ORGANIZATION_BLOCK MAIN:OB1
TITLE=Semaforo Pedonale
//Simulatore: 16
//Versione:1.0
//Data 02/03/2002
//------- Descrizione dell'impianto -----------------
//In prossimità di un passaggio pedonale si trova un
//semaforo. Premendo uno dei pulsanti di richiesta SB1 o SB2 da
//parte dei pedoni il semaforo segnala allo scadere di tempi
//prefissati la seguente sequenza sequenza:
// - verde per auto, rosso per pedoni
// - giallo per auto, rosso per pedoni
// - rosso per auto, verde per pedoni
// - rosso per auto, rosso per pedoni
// - vede per auto, rosso per pedoni

BEGIN
NETWORK 1 //Rilevamento richiesta del verde per i pedoni
//
LD I0.0
O I0.1
O M0.0
AN T35
= M0.0

NETWORK 2 //Fase del Verde per le Auto
//
LDN M0.0
ON T33
= Q0.4

NETWORK 3 //Timer per fase giallo auto
//
LD M0.0
TON T33 +50

NETWORK 4 //Fase del Giallo per le Auto
//
LD M0.0
AN T33
= Q0.3

NETWORK 5 //Fase del Rosso per le Auto
//
LD M0.0
A T33
= Q0.2

NETWORK 6 //Avvio timer per fase Verde pedoni
//
LD Q0.2
TON T34 +100

NETWORK 7 //Fase Verde per Pedoni
//
LD Q0.2
AN T34
= Q0.1

NETWORK 8 //Avvio Timer per ritardo fase giallo per le auto
//
LD M0.0
A T34
TON T35 +50

NETWORK 9 //Fase del Rosso per i pedoni
//
LD M0.0
LDN T33
O T34
ALD
ON M0.0
= Q0.0

END_ORGANIZATION_BLOCK

